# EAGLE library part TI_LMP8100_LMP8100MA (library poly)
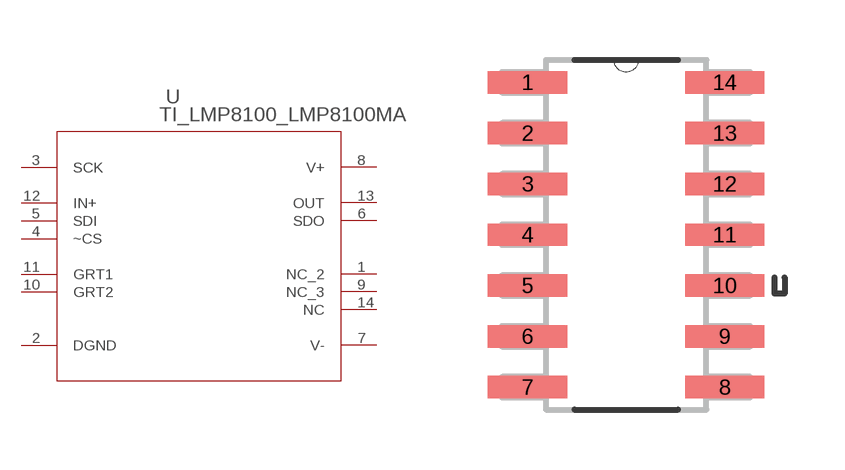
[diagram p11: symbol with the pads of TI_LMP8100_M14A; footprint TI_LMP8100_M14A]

Designator prefix U

## TI_LMP8100_LMP8100MA  [TI_LMP8100_M14A]
1  NC_2  pas
2  DGND  pas
3  SCK  in
4  ~CS  in
5  SDI  in
6  SDO  out
7  V-  pwr
8  V+  pwr
9  NC_3  pas
10  GRT2  pas
11  GRT1  pas
12  IN+  in
13  OUT  pas
14  NC  pas

## Footprint TI_LMP8100_M14A (pad centres in mm)
smd 1.981 x 0.559: 1 -2.464,3.81; 2 -2.464,2.54; 3 -2.464,1.27; 4 -2.464,0; 5 -2.464,-1.27; 6 -2.464,-2.54; 7 -2.464,-3.81; 8 2.464,-3.81; 9 2.464,-2.54; 10 2.464,-1.27; 11 2.464,0; 12 2.464,1.27; 13 2.464,2.54; 14 2.464,3.81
